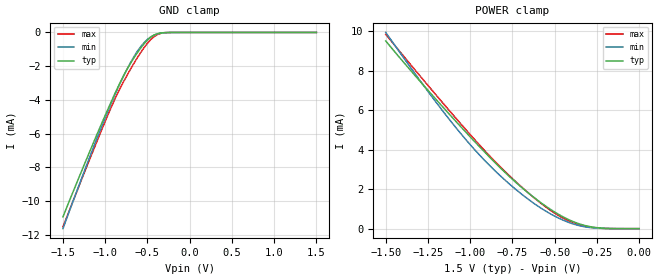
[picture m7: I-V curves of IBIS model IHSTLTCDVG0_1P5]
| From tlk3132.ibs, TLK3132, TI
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[Model]   IHSTLTCDVG0_1P5
Model_type   Input
Polarity   Non-Inverting
Vinl =   0.5500V
Vinh =   0.9500V
C_comp   0.7726pF   0.7726pF   0.7726pF
[Temperature Range]   25.0000   0.1250k   -40.0000
[Pullup Reference]   1.5000V   1.3500V   1.6500V
[Pulldown Reference]   0.000V   0.000V   0.000V
[POWER Clamp Reference]   1.5000V   1.3500V   1.6500V
[GND Clamp Reference]   0.000V   0.000V   0.000V
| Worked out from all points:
|   GND clamp passes 1 mA (typ) near -0.59 V on its own axis
|   POWER clamp passes 1 mA (typ) near -0.53 V on its own axis
[GND_clamp]
| voltage   I(typ)   I(min)   I(max)
-1.5V     -10.93mA   -11.62mA   -11.51mA
-1.14V    -6.546mA   -6.819mA   -6.979mA
-980mV    -4.685mA   -4.811mA   -5.033mA
-860mV    -3.356mA   -3.413mA   -3.679mA
-780mV    -2.541mA   -2.557mA   -2.896mA
-660mV    -1.508mA   -1.436mA   -1.832mA
-580mV    -926.9uA   -844.4uA   -1.192mA
-500mV    -456.1uA   -411.9uA   -642.8uA
-420mV    -152.4uA   -150.2uA   -245.1uA
-380mV    -72.61uA   -79.91uA   -122.7uA
-300mV    -11.9uA    -18.55uA   -18.16uA
1.5V      29.8nA     2.313uA    44.67nA
[POWER_clamp]
| voltage   I(typ)   I(min)   I(max)
-1.5V     9.511mA    9.944mA    9.848mA
-1.24V    6.913mA    6.84mA     7.156mA
-1.04V    5.019mA    4.656mA    5.157mA
-940mV    4.108mA    3.688mA    4.195mA
-860mV    3.406mA    2.99mA     3.46mA
-680mV    1.977mA    1.643mA    1.992mA
-520mV    951.9uA    726.6uA    899.5uA
-440mV    551.4uA    394.8uA    485.9uA
-380mV    320.5uA    210.9uA    262.8uA
-320mV    157.4uA    90.52uA    120.5uA
-240mV    40.51uA    19.67uA    29.83uA
0V        29.8nA     55.95nA    105.3nA
